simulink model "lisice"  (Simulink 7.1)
settings: Solver=ode45  StartTime=0.0  StopTime=10  MaxStep=0.1  RelTol=1e-3  AbsTol=1e-3
libraries: simulink x1

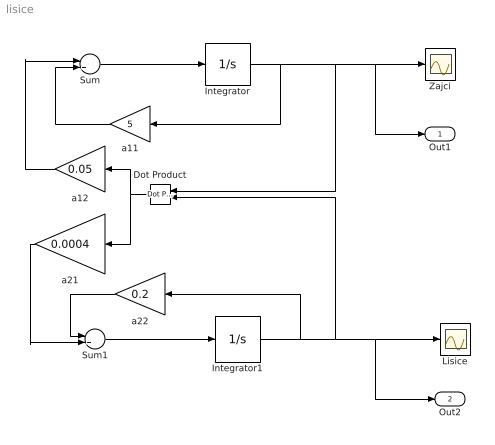
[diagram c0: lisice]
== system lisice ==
  Dot Product : simulink/Math Operations/Dot Product  Orientation=left  InputSameDT=on  OutDataType=sfix(16)  OutScaling=2^-10  DoSatur=off
  Integrator : Integrator  InitialCondition=520
  Integrator1 : Integrator  InitialCondition=85
  Lisice : Scope
  Sum : Sum  Inputs=-+  OutDataType=sfix(16)  OutScaling=2^0
  Sum1 : Sum  Inputs=-+  OutDataType=sfix(16)  OutScaling=2^0
  Zajci : Scope
  a11 : Gain  Orientation=left  Gain=5  ParameterDataType=sfix(16)  ParameterScaling=2^0  OutDataType=sfix(16)  OutScaling=2^0
  a12 : Gain  Orientation=left  Gain=0.05  ParameterDataType=sfix(16)  ParameterScaling=2^0  OutDataType=sfix(16)  OutScaling=2^0
  a21 : Gain  Orientation=left  Gain=0.0004  ParameterDataType=sfix(16)  ParameterScaling=2^0  OutDataType=sfix(16)  OutScaling=2^0
  a22 : Gain  Orientation=left  Gain=0.2  ParameterDataType=sfix(16)  ParameterScaling=2^0  OutDataType=sfix(16)  OutScaling=2^0
  Out1 : Outport  OutDataType=sfix(16)  OutScaling=2^0
  Out2 : Outport  Port=2  OutDataType=sfix(16)  OutScaling=2^0
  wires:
  Sum/1 -> Integrator/1
  Sum1/1 -> Integrator1/1
  Integrator/1 -> a11/1, Dot Product/1, Zajci/1, Out1/1
  Integrator1/1 -> a22/1, Dot Product/2, Lisice/1, Out2/1
  a22/1 -> Sum1/1
  a11/1 -> Sum/2
  a12/1 -> Sum/1
  Dot Product/1 -> a12/1, a21/1
  a21/1 -> Sum1/2
